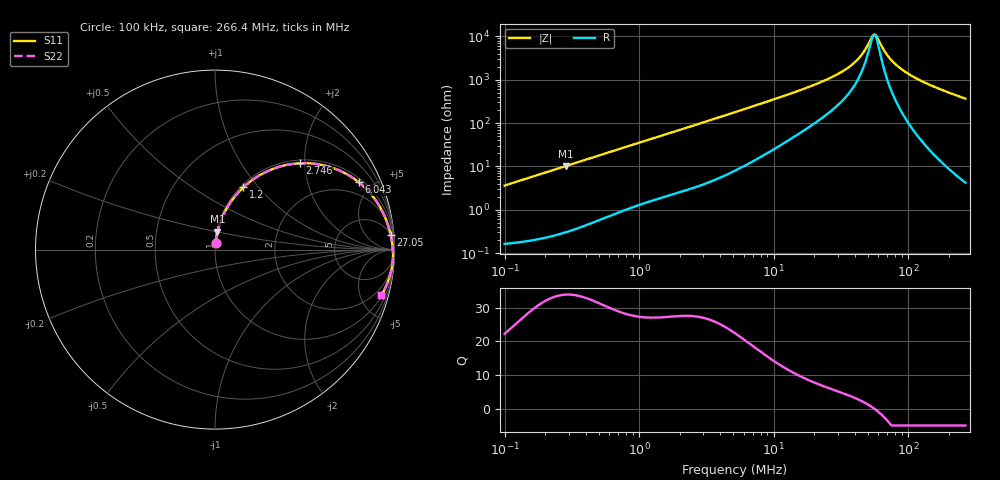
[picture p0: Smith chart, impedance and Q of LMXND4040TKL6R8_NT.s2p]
! LMXND4040TKL6R8_NT  S-PARAMETER MODEL  ( Standard Model )
! Model Generated by TAIYO YUDEN Corporation (https://www.yuden.co.jp/en/)
! Version 1.0
! TAIYO YUDEN Control No. 20251120
! Copyright(c) 2025 TAIYO YUDEN CO.,LTD. All Rights Reserved.
! Product Description (link to TY-COMPAS)
! https://ds.yuden.co.jp/TYCOMPAS/or/detail?pn=LMXND4040TKL6R8MNT&u=M
! Products Name : Inductors
! Characteristics :
!  Inductance : 6.8 [uH] , SRF(min) : 30 [MHz] , DC Resistance(max) : 0.118 [Ohm]
!  Rated Current : Saturation  1600 [mA] , Temp Rise  1860 [mA] (40 [degC])
!  Case Size : 4.0 x 4.0 / 0.157 x 0.157 [mm/inch] , Thickness : 1.8 / 0.071 [mm/inch]
!  (Conditions: Temperature = 25 [degC] , DC Bias Current = 0 [A])
! External Node Assignments :
!  1  o---GGG---o  2
! GND o---------o GND
! Frequency Range : 0.1MHz  -  266.375554MHz  [ 402 STEP ]
# MHz S RI R 50
! Freq[MHz].  S11 Real  S11 Imag  S21 Real  S21 Imag  S12 Real  S12 Imag  S22 Real  S22 Imag
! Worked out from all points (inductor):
!   401 points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, 100 kHz to 266.4 MHz, reference 50 ohm
!   read as one part in series: L = 5.74 uH near 104 kHz
!   highest Q = 33.9 at 284.4 kHz (marker M1), where L = 5.71 uH
!   self-resonance near 55 MHz
!   S11 on the Smith chart (normalised r, x): 100 kHz: 1.00, +0.07; 1.2 MHz: 1.03, +0.84; 2.746 MHz: 1.07, +1.89; 6.043 MHz: 1.20, +4.16; 27.05 MHz: 5, +22; 266.4 MHz: 1.08, -7.29
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0.1  0.00292 0.0359  0.9971 -0.0359  0.9971 -0.0359  0.00292 0.0359
0.284366  0.0132 0.1003  0.9868 -0.1003  0.9868 -0.1003  0.0132 0.1003
0.374775  0.0215 0.1306  0.9785 -0.1306  0.9785 -0.1306  0.0215 0.1306
0.718412  0.0679 0.2347  0.9321 -0.2347  0.9321 -0.2347  0.0679 0.2347
1.199584  0.1584 0.3471  0.8416 -0.3471  0.8416 -0.3471  0.1584 0.3471
1.404561  0.2016 0.3831  0.7984 -0.3831  0.7984 -0.3831  0.2016 0.3831
2.746045  0.4731 0.4813  0.5269 -0.4813  0.5269 -0.4813  0.4731 0.4813
5.26394  0.7569 0.407  0.2431 -0.407  0.2431 -0.407  0.7569 0.407
6.043062  0.8014 0.3752  0.1986 -0.3752  0.1986 -0.3752  0.8014 0.3752
10.09053  0.9105 0.2522  0.0895 -0.2522  0.0895 -0.2522  0.9105 0.2522
19.34272  0.9659 0.1296  0.0341 -0.1296  0.0341 -0.1296  0.9659 0.1296
27.04587  0.9782 0.0832  0.0218 -0.0832  0.0218 -0.0832  0.9782 0.0832
34.26619  0.984 0.0548  0.016 -0.0548  0.016 -0.0548  0.984 0.0548
40.92036  0.9872 0.0347  0.0128 -0.0347  0.0128 -0.0347  0.9872 0.0347
46.05978  0.989 0.0216  0.011 -0.0216  0.011 -0.0216  0.989 0.0216
53.93017  0.9907 0.00404  0.00931 -0.00404  0.00931 -0.00404  0.9907 0.00404
56.09953  0.991 -0.000385  0.00898 0.000385  0.00898 0.000385  0.991 -0.000385
58.35616  0.9913 -0.00484  0.0087 0.00484  0.0087 0.00484  0.9913 -0.00484
72.49162  0.992 -0.0301  0.00804 0.0301  0.00804 0.0301  0.992 -0.0301
88.29277  0.991 -0.0548  0.00899 0.0548  0.00899 0.0548  0.991 -0.0548
114.0916  0.9869 -0.0904  0.0131 0.0904  0.0131 0.0904  0.9869 -0.0904
266.3756  0.9275 -0.2536  0.0725 0.2536  0.0725 0.2536  0.9275 -0.2536
